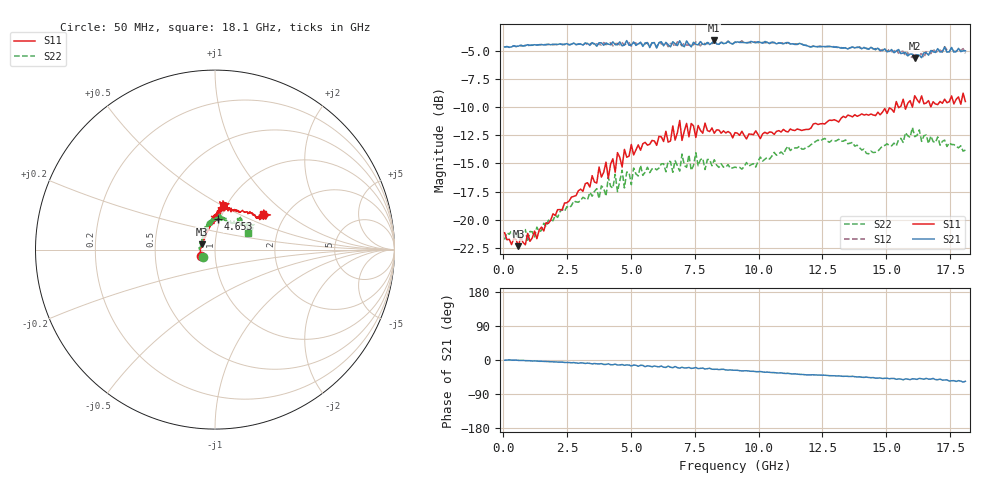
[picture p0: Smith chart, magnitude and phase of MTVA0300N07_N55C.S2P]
! Network Analyzer HP8720D.06.14 Serial No. US36140669
! 27 Jun 2005  12:07:47
! Frequency  S11  S21  S12  S22
# HZ  S  DB R 50
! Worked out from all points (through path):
!   201 points, 50 MHz to 18.1 GHz, reference 50 ohm
!   highest |S21| = -4.11 dB at 8.263 GHz (marker M1); lowest = -5.7 dB at 16.11 GHz (marker M2)
!   group delay of S21, straight-line fit = 9.06 ps
!   lowest |S11| = -22.3 dB at 591.5 MHz (marker M3), VSWR 1.17, Z = 43.3 + j2.56 ohm
!   |S11| at or under -10 dB: start of sweep to 15.35 GHz; 15.47224 GHz to 15.52879 GHz (56.55 MHz wide, 0.365 % of centre); 15.73294 GHz to 15.78822 GHz (55.29 MHz wide, 0.351 % of centre)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
!   |S22| runs from -21.9 to -11.8 dB; largest |S21 - S12| = 0.034
!   S11 on the Smith chart (normalised r, x): 50 MHz: 0.85, -0.06; 4.653 GHz: 0.98, +0.34; 18.1 GHz: 1.55, +0.69
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5e7  -21.16 -156.8  -4.68 -0.5  -4.70 -0.3  -21.77 -148.5
5.915e8  -22.34 157.4  -4.61 -1.0  -4.57 -0.9  -21.01 165.2
9.525e8  -21.21 145.0  -4.48 -1.7  -4.56 -1.5  -21.95 153.8
3.1185e9  -17.48 101.2  -4.52 -8.0  -4.51 -8.5  -18.01 116.7
4.021e9  -14.90 93.4  -4.33 -11.6  -4.48 -10.4  -17.92 106.5
4.382e9  -15.79 89.5  -4.48 -10.9  -4.39 -12.8  -15.97 104.9
4.47225e9  -14.05 84.1  -4.50 -13.3  -4.37 -11.3  -17.51 108.4
4.65275e9  -15.32 84.1  -4.59 -11.9  -4.30 -13.3  -15.62 106.1
4.743e9  -13.76 86.3  -4.51 -14.0  -4.50 -12.5  -17.19 102.0
5.104e9  -14.25 87.9  -4.23 -13.5  -4.31 -14.9  -15.42 96.3
6.09675e9  -12.61 80.6  -4.30 -18.1  -4.24 -17.5  -15.42 90.1
6.63825e9  -11.68 80.3  -4.22 -20.2  -4.37 -18.3  -15.79 85.1
6.7285e9  -12.94 84.6  -4.39 -17.2  -4.66 -18.8  -14.76 82.3
6.909e9  -11.20 80.7  -4.13 -21.3  -4.35 -19.3  -15.69 81.2
6.99925e9  -12.97 80.5  -4.51 -19.1  -4.60 -21.6  -14.18 81.5
7.17975e9  -11.46 84.4  -4.14 -20.9  -4.51 -19.8  -15.36 76.1
8.26275e9  -12.34 78.2  -4.11 -24.6  -4.33 -25.3  -14.68 70.5
9.075e9  -12.28 74.8  -4.27 -26.9  -4.24 -27.0  -15.33 66.0
1.21435e10  -11.51 54.9  -4.62 -39.1  -4.58 -39.2  -13.20 53.1
1.512175e10  -10.09 33.9  -5.07 -49.6  -4.86 -49.1  -13.43 40.2
1.61145e10  -9.00 33.4  -5.67 -50.1  -5.22 -50.2  -12.64 35.2
1.81e10  -9.52 36.4  -5.02 -56.1  -5.24 -56.6  -13.83 27.0
